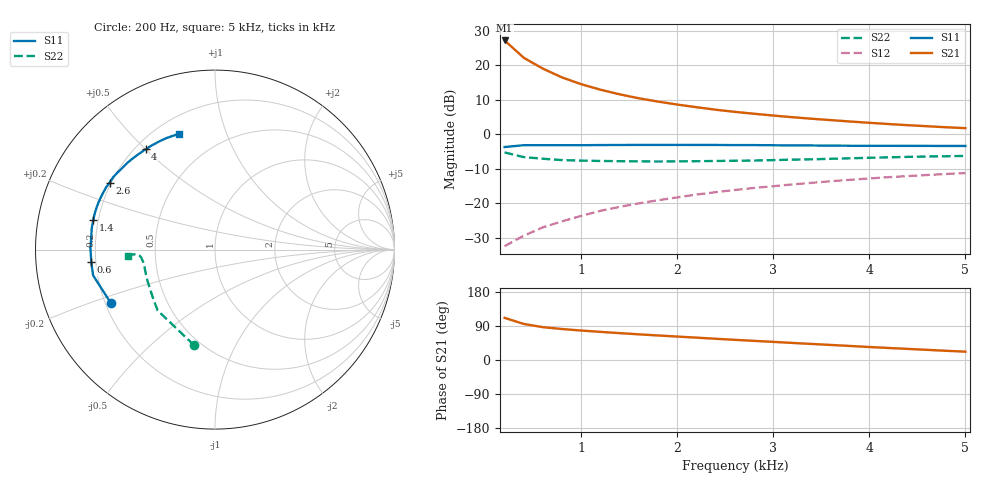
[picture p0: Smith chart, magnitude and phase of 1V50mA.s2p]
#  HZ  S  MA  R  50.0000
! Device:MCH4020
! Bias:VCE=1V, IC=50mA
!MHZ	S11(MAG/ANG)		S21(MAG/ANG)		S12(MAG/ANG)		S22(MAG/ANG)
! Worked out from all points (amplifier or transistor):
!   25 points, 200 Hz to 5 kHz, reference 50 ohm
!   highest |S21| = 27.1 dB at 200 Hz (marker M1)
!   |S21| within 3 dB of that: start of sweep to 319.5 Hz
!   unconditionally stable (mu >= 1): 1.522 kHz to end of sweep
!   at 1 kHz: K = 0.94, MSG = 19.0 dB, |S12| = -23.6 dB
!   at 2.6 kHz: K = 1.03, MAG = 10.2 dB, |S12| = -16.1 dB
!   at 5 kHz: K = 1.00, MAG = 6.1 dB, |S12| = -11.2 dB
!   S11 on the Smith chart (normalised r, x): 200 Hz: 0.22, -0.23; 600 Hz: 0.18, -0.05; 1.4 kHz: 0.18, +0.12; 2.6 kHz: 0.19, +0.28; 4 kHz: 0.24, +0.50; 5 kHz: 0.29, +0.69
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200  0.652 -152.6  22.72 111.2  0.024 50.4  0.545 -102.4
400  0.694 -168.0  12.74 95.1  0.034 54.6  0.466 -133.3
600  0.693 -174.1  8.865 86.6  0.045 58.6  0.442 -140.7
800  0.694 179.3  6.618 81.7  0.055 61.5  0.422 -149.5
1000  0.693 174.3  5.279 77.7  0.066 63.1  0.415 -154.8
1200  0.697 170.1  4.399 74.2  0.078 64.0  0.41 -159.2
1400  0.698 166.3  3.771 70.8  0.089 64.0  0.407 -162.2
1600  0.7 162.8  3.307 67.7  0.1 63.8  0.405 -165.0
1800  0.7 159.6  2.961 64.7  0.111 63.3  0.403 -167.1
2000  0.7 156.8  2.683 61.8  0.122 62.7  0.405 -169.1
2200  0.699 153.5  2.457 59.0  0.134 61.8  0.407 -170.8
2400  0.699 150.5  2.26 56.0  0.145 60.6  0.41 -172.2
2600  0.696 147.6  2.105 53.2  0.156 59.4  0.413 -173.6
2800  0.696 144.6  1.976 50.5  0.167 58.2  0.416 -174.4
3000  0.692 141.5  1.861 47.8  0.177 56.8  0.422 -175.4
3200  0.688 138.3  1.761 45.0  0.188 55.4  0.429 -175.9
3400  0.687 135.0  1.674 42.3  0.198 53.8  0.433 -176.3
3800  0.681 128.3  1.526 37.0  0.219 50.8  0.448 -176.6
4000  0.68 124.7  1.462 34.3  0.229 49.2  0.456 -176.6
4200  0.679 121.2  1.403 31.7  0.239 47.5  0.463 -176.6
4800  0.676 110.7  1.26 24.3  0.266 42.5  0.48 -176.1
5000  0.676 107.4  1.224 22.0  0.274 40.9  0.485 -176.0
